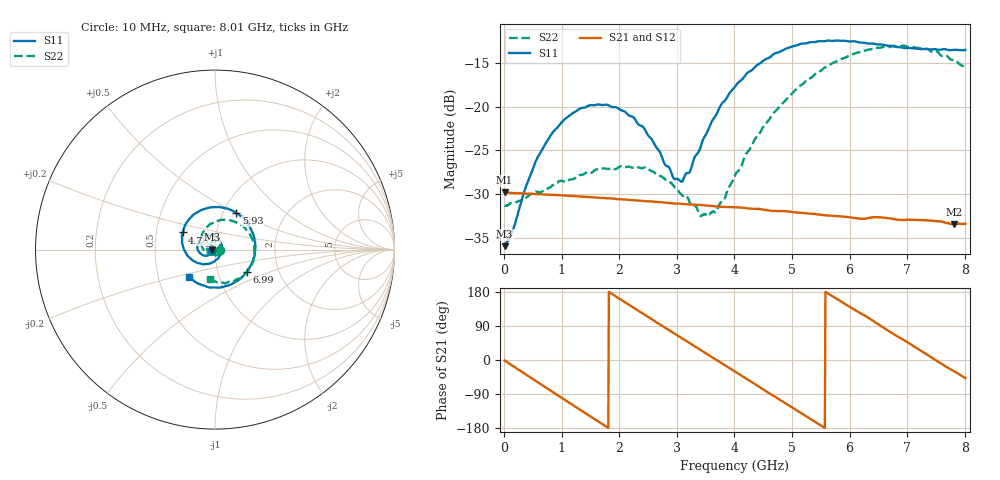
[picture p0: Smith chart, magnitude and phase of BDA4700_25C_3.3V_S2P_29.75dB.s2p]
!Agilent Technologies,E5071B,MY42404982,A.09.10
!Date: Mon Oct 20 18:15:35 2025
!Data & Calibration Information:
!Freq	S11:SOLT2(ON)	S21:SOLT2(ON)	S12:SOLT2(ON)	S22:SOLT2(ON)
# Hz S RI R 50
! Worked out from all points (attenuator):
!   801 points, 10 MHz to 8.01 GHz, reference 50 ohm
!   highest |S21| = -29.80 dB at 10 MHz (marker M1); lowest = -33.4 dB at 7.81 GHz (marker M2)
!   lowest |S11| = -35.9 dB at 10 MHz (marker M3), VSWR 1.03, Z = 48.4 - j0.115 ohm
!   |S11| at or under -10 dB: start of sweep to end of sweep
!   |S22| runs from -32.5 to -13.0 dB; largest |S21 - S12| = 0.00035
!   S11 on the Smith chart (normalised r, x): 10 MHz: 0.97, -0.00; 4.76 GHz: 0.68, +0.14; 5.93 GHz: 1.15, +0.50; 6.99 GHz: 1.38, -0.36; 8.01 GHz: 0.71, -0.23
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1e7  -0.0159 -0.00118  0.0323 -0.000672  0.0324 -0.000706  0.0272 -0.000818
1.5e8  -0.017 -0.00981  0.0309 -0.00848  0.0309 -0.00849  0.0273 -0.00731
6e8  -0.0405 -0.0334  0.0157 -0.0274  0.0157 -0.0274  0.0132 -0.0296
1.01e9  -0.0785 -0.0246  -0.00577 -0.0305  -0.00576 -0.0306  -0.0152 -0.0345
1.35e9  -0.0982 0.00701  -0.0213 -0.0219  -0.0214 -0.022  -0.0364 -0.0183
2.08e9  -0.05 0.08  -0.0266 0.0127  -0.0266 0.0127  -0.0303 0.0336
2.68e9  0.0266 0.0498  -0.00317 0.0283  -0.00324 0.0283  0.0126 0.0384
2.95e9  0.0376 0.00938  0.00927 0.0264  0.00924 0.0263  0.0255 0.0241
3.09e9  0.0349 -0.0132  0.0151 0.0234  0.0149 0.0234  0.0283 0.013
3.41e9  0.00459 -0.0582  0.0245 0.0123  0.0245 0.0124  0.0212 -0.0107
3.55e9  -0.0176 -0.0723  0.0265 0.00625  0.0265 0.00621  0.0131 -0.0199
3.7e9  -0.0465 -0.0794  0.0269 -0.000402  0.0269 -0.00049  0.000455 -0.0257
4.01e9  -0.1108 -0.068  0.0229 -0.0135  0.023 -0.0134  -0.0309 -0.0259
4.76e9  -0.1804 0.0954  -0.00535 -0.0247  -0.00518 -0.0248  -0.0781 0.0591
5.35e9  -0.0659 0.2242  -0.0228 -0.00896  -0.0227 -0.00906  -0.0158 0.1465
5.93e9  0.119 0.2054  -0.0196 0.0129  -0.0197 0.0128  0.1138 0.1531
6.35e9  0.2087 0.0942  -0.00753 0.0219  -0.00753 0.0218  0.1942 0.0854
6.68e9  0.2216 -0.0217  0.00539 0.0224  0.00551 0.0224  0.2192 0.000643
6.99e9  0.1773 -0.1231  0.0151 0.0168  0.0152 0.0167  0.2047 -0.0815
7.44e9  0.0418 -0.2084  0.0222 0.00186  0.0223 0.00193  0.1162 -0.1679
7.81e9  -0.0898 -0.1909  0.0185 -0.0104  0.0186 -0.0105  0.0182 -0.1837
8.01e9  -0.1473 -0.1507  0.0143 -0.0159  0.0143 -0.0159  -0.0295 -0.1633
